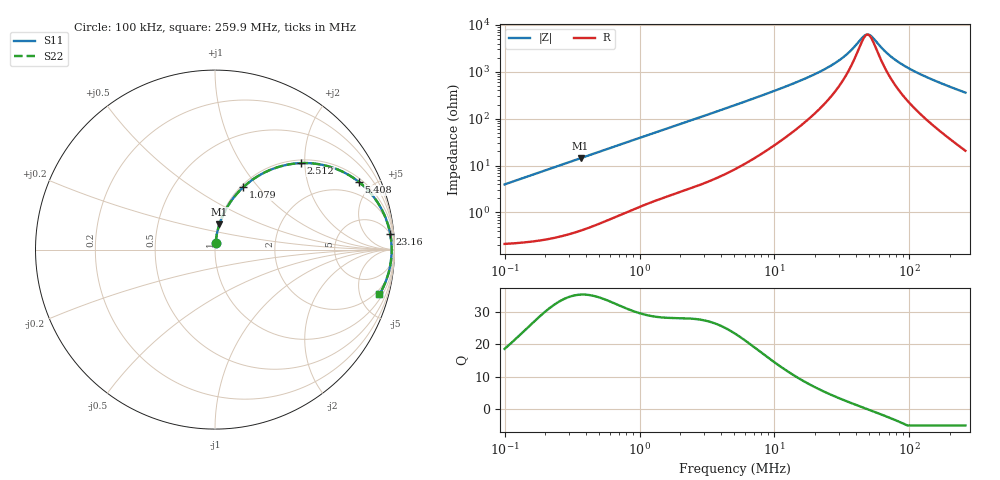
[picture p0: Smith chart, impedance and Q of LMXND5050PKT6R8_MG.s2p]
! LMXND5050PKT6R8_MG  S-PARAMETER MODEL  ( General Type )
! Model Generated by TAIYO YUDEN Corporation (http://www.ty-top.com)
! Version 1.0
! TAIYO YUDEN Control No. 191023NI43SB-FBB
! Copyright(c) 2019 TAIYO YUDEN CO.,LTD. All Rights Reserved.
! Product Description (link to TY-COMPAS)
! https://ds.yuden.co.jp/TYCOMPAS/or/detail?pn=LMXND5050PKT6R8MMG&u=M
! Products Name : Inductors
! Characteristics :
!  Inductance : 6.8 uH , SRF(min) : 33 MHz , DC Resistance(max) : 0.18 Ohm
!  Rated Current : Saturation :1600 mA , Temp Rise : 1200 mA
!  Case Size : 4.9 x 4.9 / 0.193 x 0.193 [mm/inch] , Thickness : 1.4 / 0.055 [mm/inch]
!  (Conditions: Temperature = 25 degC , DC Bias Current/Voltage = 0A / 0V)
! External Node Assignments :
!  1  o---GGG---o  2
! GND o---------o GND
! Frequency Range : 0.1MHz  -  259.929867MHz  [ 402 STEP ]
# MHz S RI R 50
! Freq[MHz].  S11 Real  S11 Imag  S21 Real  S21 Imag  S12 Real  S12 Imag  S22 Real  S22 Imag
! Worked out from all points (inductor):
!   401 points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, 100 kHz to 259.9 MHz, reference 50 ohm
!   read as one part in series: L = 6.3 uH near 104 kHz
!   highest Q = 35.3 at 366 kHz (marker M1), where L = 6.27 uH
!   self-resonance near 48.93 MHz
!   S11 on the Smith chart (normalised r, x): 100 kHz: 1.00, +0.08; 1.079 MHz: 1.03, +0.84; 2.512 MHz: 1.07, +1.92; 5.408 MHz: 1.18, +4.14; 23.16 MHz: 5, +22; 259.9 MHz: 1.41, -7.19
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0.1  0.00368 0.0394  0.9963 -0.0394  0.9963 -0.0394  0.00368 0.0394
0.365975  0.0242 0.1402  0.9758 -0.1402  0.9758 -0.1402  0.0242 0.1402
0.37324  0.0251 0.1428  0.9749 -0.1428  0.9749 -0.1428  0.0251 0.1428
0.673136  0.0715 0.2427  0.9285 -0.2427  0.9285 -0.2427  0.0715 0.2427
1.078932  0.1576 0.3476  0.8424 -0.3476  0.8424 -0.3476  0.1576 0.3476
1.393082  0.2321 0.4049  0.7679 -0.4049  0.7679 -0.4049  0.2321 0.4049
2.512413  0.4804 0.482  0.5196 -0.482  0.5196 -0.482  0.4804 0.482
3.509316  0.637 0.4625  0.363 -0.4625  0.363 -0.4625  0.637 0.4625
5.098332  0.7821 0.3919  0.2179 -0.3919  0.2179 -0.3919  0.7821 0.3919
5.408035  0.8006 0.3781  0.1994 -0.3781  0.1994 -0.3781  0.8006 0.3781
9.377335  0.9172 0.2448  0.0828 -0.2448  0.0828 -0.2448  0.9172 0.2448
19.02902  0.9708 0.1128  0.0292 -0.1128  0.0292 -0.1128  0.9708 0.1128
23.16263  0.9766 0.0852  0.0234 -0.0852  0.0234 -0.0852  0.9766 0.0852
32.99563  0.9824 0.0423  0.0176 -0.0423  0.0176 -0.0423  0.9824 0.0423
45.19087  0.9842 0.00833  0.0158 -0.00833  0.0158 -0.00833  0.9842 0.00833
47.93603  0.9843 0.00214  0.0157 -0.00214  0.0157 -0.00214  0.9843 0.00214
49.85818  0.9843 -0.00198  0.0157 0.00198  0.0157 0.00198  0.9843 -0.00198
52.88686  0.9843 -0.00817  0.0157 0.00817  0.0157 0.00817  0.9843 -0.00817
71.02397  0.9827 -0.0399  0.0173 0.0399  0.0173 0.0399  0.9827 -0.0399
88.1685  0.98 -0.0651  0.02 0.0651  0.02 0.0651  0.98 -0.0651
116.1003  0.9738 -0.1012  0.0262 0.1012  0.0262 0.1012  0.9738 -0.1012
259.9299  0.916 -0.25  0.084 0.25  0.084 0.25  0.916 -0.25
